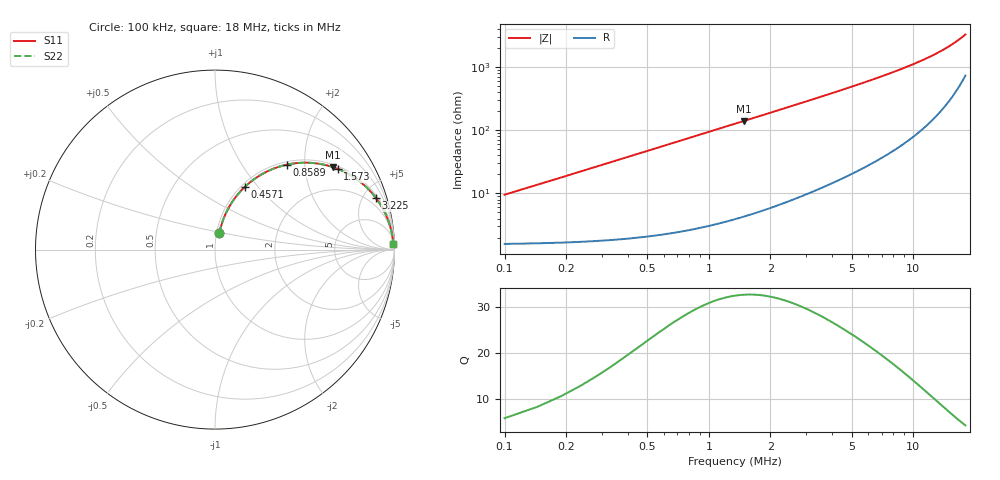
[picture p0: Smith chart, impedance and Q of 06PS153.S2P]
! Coilcraft 0603PS-153 Power Chip Inductor
! 19 February 2003
# MHZ S MA R 50
!Freq  MagS11  AngS11  MagS21  AngS21  MagS12  AngS12  MagS22  AngS22
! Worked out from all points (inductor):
!   402 points, 100 kHz to 18 MHz, reference 50 ohm
!   read as one part in series: L = 15 uH near 189.3 kHz
!   highest Q = 32.6 at 1.484 MHz (marker M1), where L = 15 uH
!   S11 on the Smith chart (normalised r, x): 100 kHz: 1.03, +0.19; 457.1 kHz: 1.04, +0.86; 858.9 kHz: 1.06, +1.62; 1.573 MHz: 1.09, +2.98; 3.225 MHz: 1.21, +6.17; 18 MHz: 16, +64
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0.1  0.09368 75.1  0.9801 -5.3  0.9801 -5.3  0.09368 75.1
0.14464  0.1339 75.6  0.9753 -7.6  0.9753 -7.6  0.1339 75.6
0.23392  0.2125 73.3  0.9608 -12.2  0.9608 -12.2  0.2125 73.3
0.27856  0.2504 71.7  0.9515 -14.5  0.9515 -14.5  0.2504 71.7
0.36784  0.3226 68.1  0.9292 -18.8  0.9292 -18.8  0.3226 68.1
0.45712  0.3895 64.4  0.903 -22.9  0.903 -22.9  0.3895 64.4
0.63568  0.5059 57.4  0.8433 -30.4  0.8433 -30.4  0.5059 57.4
0.85888  0.6195 49.8  0.7642 -38.3  0.7642 -38.3  0.6195 49.8
1.17136  0.7306 41.3  0.6603 -46.9  0.6603 -46.9  0.7306 41.3
1.48384  0.8028 34.9  0.5721 -53.4  0.5721 -53.4  0.8028 34.9
1.57312  0.8185 33.3  0.5499 -54.9  0.5499 -54.9  0.8185 33.3
1.8856  0.8614 28.8  0.4821 -59.4  0.4821 -59.4  0.8614 28.8
2.19808  0.891 25.3  0.4269 -62.9  0.4269 -62.9  0.891 25.3
2.59984  0.9169 21.7  0.3704 -66.4  0.3704 -66.4  0.9169 21.7
3.09088  0.9376 18.5  0.3172 -69.6  0.3172 -69.6  0.9376 18.5
3.2248  0.9419 17.7  0.305 -70.3  0.305 -70.3  0.9419 17.7
4.51936  0.9669 12.7  0.2199 -75.0  0.2199 -75.0  0.9669 12.7
6.08176  0.9795 9.3  0.1613 -78.1  0.1613 -78.1  0.9795 9.3
9.07264  0.9884 5.8  0.1011 -80.6  0.1011 -80.6  0.9884 5.8
12.06352  0.9915 3.9  0.06794 -80.9  0.06794 -80.9  0.9915 3.9
15.0544  0.9926 2.6  0.04603 -79.5  0.04603 -79.5  0.9926 2.6
18  0.9928 1.7  0.03023 -75.4  0.03023 -75.4  0.9928 1.7
